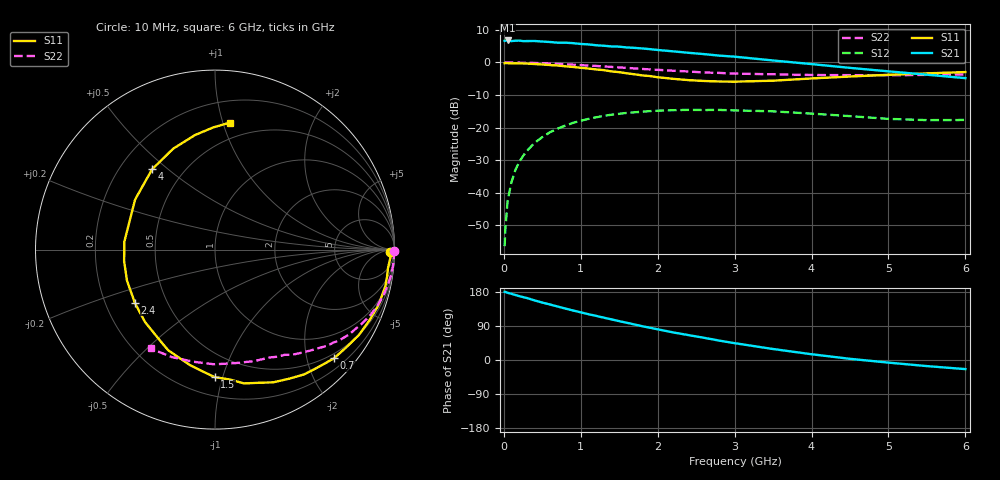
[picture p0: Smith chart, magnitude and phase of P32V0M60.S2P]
! SIEMENS Small Signal Semiconductors
! BFP181
! Si NPN RF Bipolar Junction Transistor in SOT143
! VCE = 2 V  IC = 0.6 mA
! Common Emitter S-Parameters:  March  1996
# GHz  S  MA  R  50
!  f  S11  S21  S12  S22
! GHz  MAG  ANG  MAG  ANG  MAG  ANG  MAG  ANG
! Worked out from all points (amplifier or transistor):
!   36 points, 10 MHz to 6 GHz, reference 50 ohm
!   highest |S21| = 6.8 dB at 50 MHz (marker M1)
!   |S21| within 3 dB of that: start of sweep to 2.035 GHz
!   unconditionally stable (mu >= 1): 3.587 GHz to end of sweep
!   at 250 MHz: K = 0.08, MSG = 17.7 dB, |S12| = -28.7 dB
!   at 1.4 GHz: K = 0.45, MSG = 10.5 dB, |S12| = -16.1 dB
!   at 6 GHz: K = 1.43, MAG = 2.5 dB, |S12| = -17.7 dB
!   S11 on the Smith chart (normalised r, x): 10 MHz: 62, -29; 700 MHz: 0.40, -2.52; 1.5 GHz: 0.33, -0.94; 2.4 GHz: 0.33, -0.27; 4 GHz: 0.33, +0.44; 6 GHz: 0.37, +1.06
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0.01  0.9739 -0.7  2.152 179.9  0.0015 84.4  0.9989 -0.3
0.02  0.9805 -1.4  2.165 179.6  0.0028 89.3  0.9984 -0.6
0.05  0.9781 -2.7  2.182 177.3  0.0076 90.1  0.9965 -1.5
0.1  0.9693 -6.1  2.134 174.6  0.0146 86.1  0.9973 -2.9
0.15  0.9705 -9.2  2.159 171.5  0.0222 84.3  0.9965 -4.3
0.2  0.9706 -12.3  2.172 168.6  0.0296 81.9  0.9951 -5.8
0.25  0.9651 -15.2  2.132 165.9  0.0366 79.6  0.9923 -7.3
0.4  0.9468 -24.5  2.14 157.2  0.0581 73.1  0.9829 -11.7
0.5  0.9327 -30.6  2.099 151.5  0.0713 68.8  0.9741 -14.5
0.7  0.8983 -42.4  2.017 141.1  0.0964 60.8  0.9528 -19.9
0.9  0.8543 -54.5  1.984 130.6  0.118 52.8  0.9264 -25.0
1.1  0.8076 -66.3  1.898 120.8  0.1359 45.7  0.8969 -29.8
1.5  0.7104 -90.1  1.752 102.5  0.1628 32.8  0.8384 -38.2
1.8  0.6331 -108.9  1.644 89.1  0.1752 24.7  0.7962 -43.6
2.2  0.5611 -134.1  1.484 72.8  0.1847 14.7  0.7474 -50.4
2.4  0.5358 -146.5  1.41 65.7  0.1871 10.2  0.7271 -53.7
3  0.5072 175.1  1.229 44.4  0.1835 -1.1  0.675 -62.8
3.5  0.5251 148.0  1.074 29.0  0.1775 -8.0  0.6586 -70.6
4  0.5684 128.1  0.945 15.2  0.1637 -13.2  0.6424 -80.0
4.5  0.6088 112.4  0.827 3.1  0.1498 -16.5  0.6391 -90.3
5.5  0.6805 90.9  0.649 -16.1  0.13 -12.7  0.6455 -111.9
6  0.7125 83.3  0.575 -24.0  0.1307 -9.2  0.6576 -123.1
